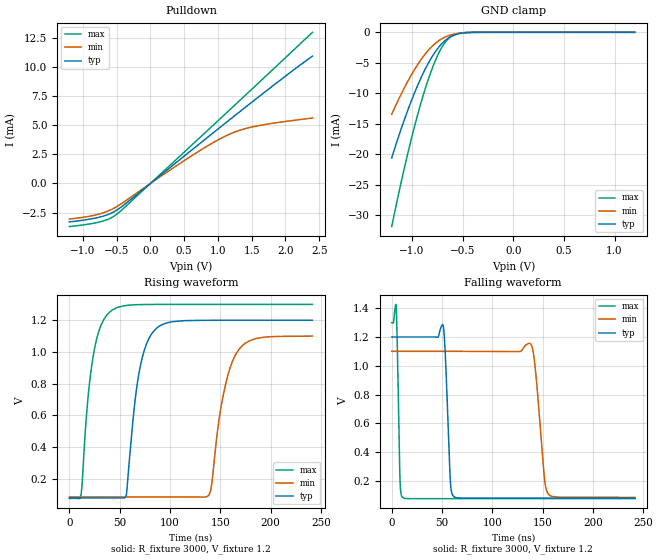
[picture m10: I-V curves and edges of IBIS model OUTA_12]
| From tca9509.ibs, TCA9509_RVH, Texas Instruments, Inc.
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[Model]   OUTA_12
Model_type  Open_drain
Enable   Active-High
Vref =   1.2
Rref =   1350
Cref =   50p
Vmeas =   0.6
| variable   typ   min   max
C_comp   2.16pF   1.49pF   2.55pF
| C_pulldown   1.46pF   1.02pF   1.68pF
| C_tri-state   2.16pF   1.49pF   2.55pF
[Temperature Range]   40   100   -40
| Ambient temperature   25   85   -40
[Voltage range]   1.2   1.1   1.3
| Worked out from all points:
|   slope of the pulldown table from 0 to 0.18 V, typ, clamps not added: 213 ohm
|   GND clamp passes 1 mA (typ) near -0.64 V on its own axis
|   rising waveform, R_fixture 3000, V_fixture 1.2: 20-80 % time 13.5ns typ, 16ns min, 12.1ns max; typ from 0.079 V to 1.2 V
|   falling waveform, R_fixture 3000, V_fixture 1.2: 20-80 % time 3.69ns typ, 7.08ns min, 2.06ns max; typ from 1.2 V to 0.079 V
[GND Clamp]
| OUTA_12
|   Voltage   I(typ)   I(min)   I(max)
-1.2V     -20.64mA   -13.47mA   -31.91mA
-1.115V   -16.28mA   -10.44mA   -25.25mA
-1.03V    -12.31mA   -7.711mA   -19.12mA
-955mV    -9.166mA   -5.595mA   -14.22mA
-880mV    -6.411mA   -3.798mA   -9.867mA
-810mV    -4.247mA   -2.449mA   -6.383mA
-745mV    -2.641mA   -1.502mA   -3.732mA
-685mV    -1.536mA   -880.7uA   -1.932mA
-625mV    -789uA     -472.8uA   -836.2uA
-550mV    -278.9uA   -190uA     -228uA
-435mV    -35.16uA   -33.42uA   -15.6uA
1.2V      399.9pA    2.186nA    66.79pA
[Pulldown]
| OUTA_12
|   Voltage   I(typ)   I(min)   I(max)
-1.2V     -3.295mA   -3.049mA   -3.694mA
-925mV    -3.084mA   -2.832mA   -3.494mA
-725mV    -2.841mA   -2.566mA   -3.26mA
-595mV    -2.584mA   -2.281mA   -2.988mA
-485mV    -2.235mA   -1.935mA   -2.574mA
595mV     2.784mA    2.313mA    3.194mA
920mV     4.293mA    3.468mA    4.94mA
1.16V     5.4mA      4.191mA    6.232mA
1.35V     6.271mA    4.608mA    7.257mA
1.57V     7.272mA    4.919mA    8.446mA
2.4V      10.92mA    5.608mA    12.95mA
[Ramp]
| OUTA_12
| variable   typ   min   max
dV/dt_r   0.67/1.35E-08   0.61/1.60E-08   0.74/1.21E-08
dV/dt_f   0.72/4.03E-09   0.64/7.53E-09   0.81/2.29E-09
R_load = 3000
[Rising Waveform]
| OUTA_12
R_fixture =   3000
C_fixture =   0
L_fixture =   0
V_fixture =   1.2
V_fixture_min = 1.1
V_fixture_max = 1.3
|   Time   V(typ)   V(min)   V(max)
0s        79.5mV     84.79mV    75.99mV
11.27ns   79.5mV     84.79mV    83.76mV
23.17ns   79.5mV     84.79mV    954.1mV
39.94ns   79.5mV     84.79mV    1.252V
56.39ns   92.33mV    84.79mV    1.293V
69.32ns   870.9mV    84.79mV    1.298V
86.4ns    1.148V     84.79mV    1.3V
139.1ns   1.2V       101.7mV    1.3V
171ns     1.2V       1.034V     1.3V
241.5ns   1.2V       1.1V       1.3V
[Falling Waveform]
| OUTA_12
R_fixture =   3000
C_fixture =   0
L_fixture =   0
V_fixture =   1.2
V_fixture_min = 1.1
V_fixture_max = 1.3
|   Time   V(typ)   V(min)   V(max)
0s        1.2V       1.1V       1.3V
4.485ns   1.2V       1.1V       1.403V
8.325ns   1.2V       1.1V       193.6mV
11.46ns   1.2V       1.1V       81.11mV
51.01ns   1.282V     1.1V       75.99mV
58.31ns   194.8mV    1.1V       75.99mV
61.96ns   88.54mV    1.1V       75.99mV
137.8ns   79.5mV     1.154V     75.99mV
155.2ns   79.5mV     110.8mV    75.99mV
241.5ns   79.5mV     84.79mV    75.99mV
